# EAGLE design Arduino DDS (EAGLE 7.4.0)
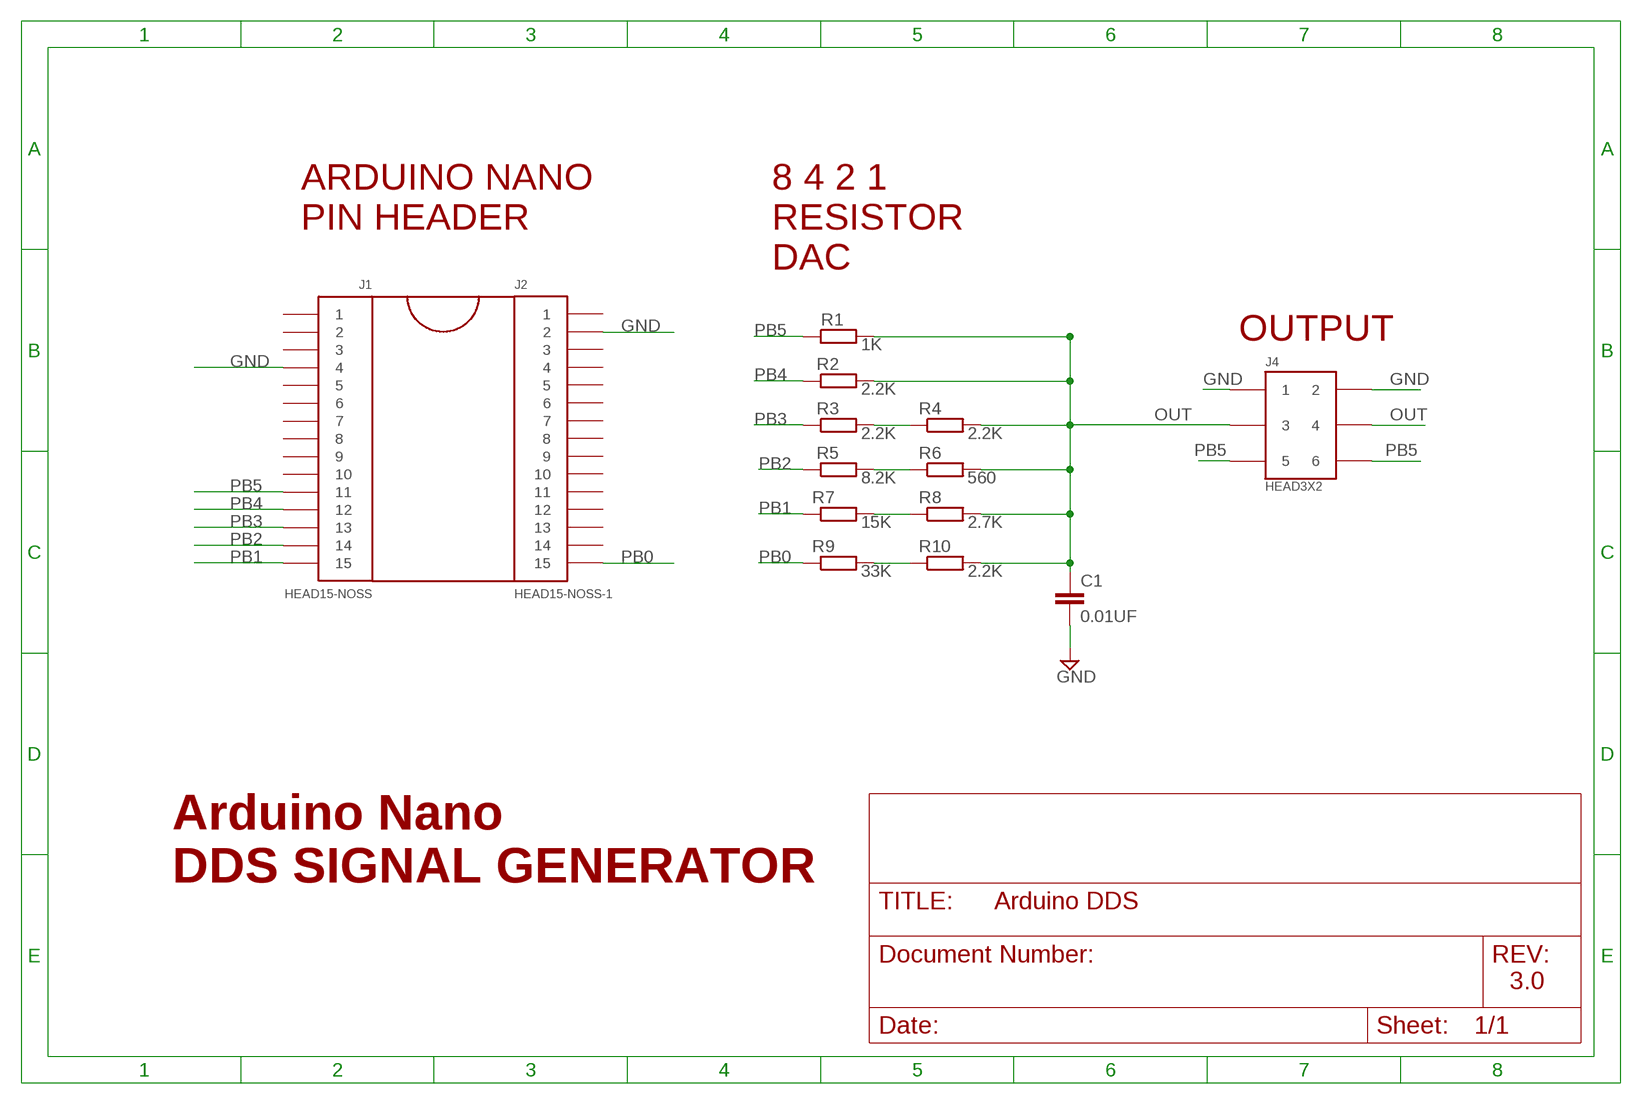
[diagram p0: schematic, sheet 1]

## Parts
C1  0.01UF  C-EUC0805  [C0805]
J1  HEAD15-NOSS  [HEAD15-NOSS]
J2  HEAD15-NOSS-1  [HEAD15-NOSS-1]
J4  HEAD3X2  [HEAD3X2]
R1  1K  R-EU_M0805  [M0805]
R2  2.2K  R-EU_M0805  [M0805]
R3  2.2K  R-EU_M0805  [M0805]
R4  2.2K  R-EU_M0805  [M0805]
R5  8.2K  R-EU_M0805  [M0805]
R6  560  R-EU_M0805  [M0805]
R7  15K  R-EU_M0805  [M0805]
R8  2.7K  R-EU_M0805  [M0805]
R9  33K  R-EU_M0805  [M0805]
R10  2.2K  R-EU_M0805  [M0805]

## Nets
GND: C1.2 J1.4 J2.2 J4.1 J4.2
N$7: R3.2 R4.1
N$8: R5.2 R6.1
N$9: R7.2 R8.1
N$10: R9.2 R10.1
OUT: C1.1 J4.3 J4.4 R1.2 R2.2 R4.2 R6.2 R8.2 R10.2
PB0: J2.15 R9.1
PB1: J1.15 R7.1
PB2: J1.14 R5.1
PB3: J1.13 R3.1
PB4: J1.12 R2.1
PB5: J1.11 J4.5 J4.6 R1.1
Unconnected: J1.1 J1.2 J1.3 J1.5 J1.6 J1.7 J1.8 J1.9 J1.10 J2.1 J2.3 J2.4 J2.5 J2.6 J2.7 J2.8 J2.9 J2.10 J2.11 J2.12 J2.13 J2.14

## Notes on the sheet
- ARDUINO NANO
  PIN HEADER
- 8 4 2 1
  RESISTOR
  DAC
- OUTPUT
- Arduino Nano
  DDS SIGNAL GENERATOR
- 3.0

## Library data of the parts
C1 = resistor:C-EU: CAPACITOR, European symbol
J1 = MyCON2:HEAD15-NOSS
J2 = MyCON2:HEAD15-NOSS-1
J4 = MyCON2:HEAD3X2
R1-R10 = resistor:R-EU_: RESISTOR, European symbol

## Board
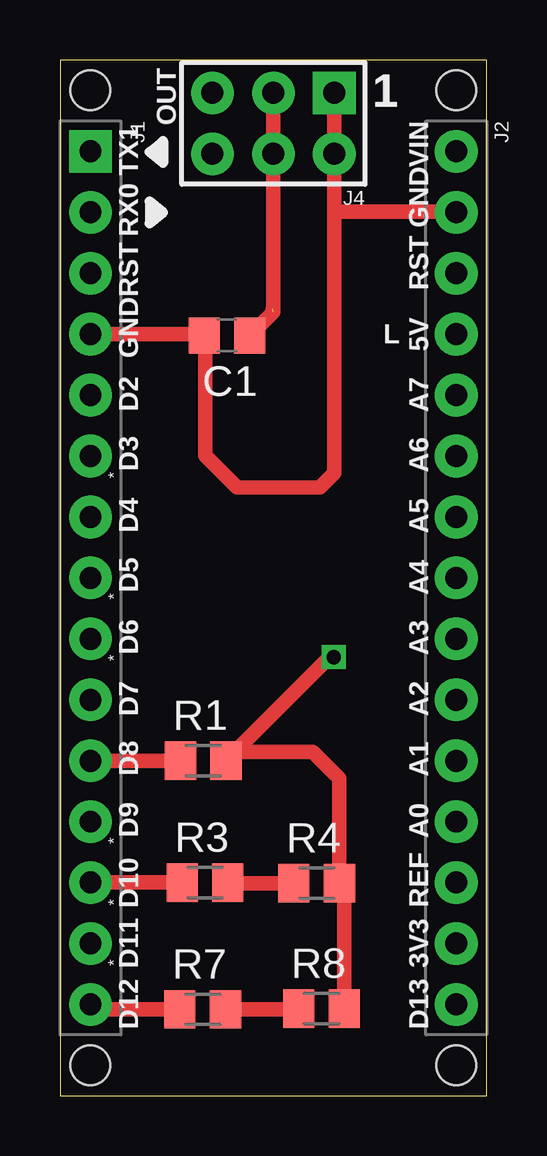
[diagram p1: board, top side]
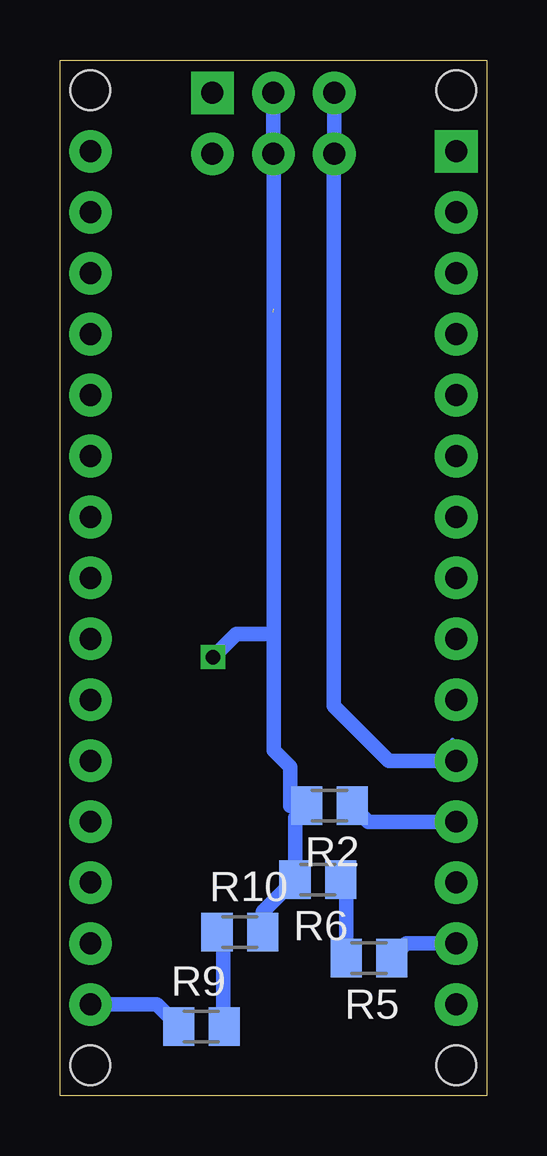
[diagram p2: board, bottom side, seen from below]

Size 17.78 x 43.18 mm. Coordinates in mm from the lower left corner, seen from the top.
Outline: 0,0 17.78,0 17.78,43.18 0,43.18 0,0
Copper layers (1*16): Top 0.035mm / dielectric 1.5mm / Bottom 0.035mm
Design rules "default *": minimum track width 8mil, minimum drill 16mil, track to track 8mil, track to pad 8mil, pad to pad 8mil, via to via 8mil, smd to smd 8mil, copper to edge 8mil, drill to drill 8mil, minimum pad ring 12mil, minimum via ring 8mil, stop-mask expansion 4mil, vias tented up to drill 18mil, thermal gap 10mil
Holes 1.65 mm at 1.27,1.27 16.51,1.27 16.51,41.91 1.27,41.91
tRestrict: area 0.1,0.1 to 2.4,2.4; area 15.4,40.8 to 17.7,43.1; area 15.4,0.1 to 17.7,2.4; area 0.1,40.8 to 2.4,43.1
bRestrict: area 15.4,0.1 to 17.7,2.4; area 0.1,0.1 to 2.4,2.4; area 0.1,40.8 to 2.4,43.1; area 15.4,40.8 to 17.7,43.1

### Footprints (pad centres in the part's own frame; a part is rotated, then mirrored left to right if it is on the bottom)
C0805 = smd 1.3 x 1.5: 1 -0.95,0; 2 0.95,0
HEAD15-NOSS = drill 0.914 pad 1.778 square: 1 0,0 | drill 0.914 pad 1.778: 2 2.54,0; 3 5.08,0; 4 7.62,0; 5 10.16,0; 6 12.7,0; 7 15.24,0; 8 17.78,0; 9 20.32,0; 10 22.86,0; 11 25.4,0; 12 27.94,0; 13 30.48,0; 14 33.02,0; 15 35.56,0
HEAD15-NOSS-1 = drill 0.914 pad 1.778: 1 0,0; 2 2.54,0; 3 5.08,0; 4 7.62,0; 5 10.16,0; 6 12.7,0; 7 15.24,0; 8 17.78,0; 9 20.32,0; 10 22.86,0; 11 25.4,0; 12 27.94,0; 13 30.48,0; 14 33.02,0; 15 35.56,0
HEAD3X2 = drill 0.914 pad 1.778 square: 1 0,0 | drill 0.914 pad 1.778: 2 0,2.54; 3 2.54,0; 4 2.54,2.54; 5 5.08,0; 6 5.08,2.54
M0805 = smd 1.3 x 1.6: 1 -0.95,0; 2 0.95,0

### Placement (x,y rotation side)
C1  6.96,31.7 180 top
J1  1.27,39.37 270 top
J2  16.51,39.37 270 top
J4  11.43,41.81 180 top
R1  5.97,13.97 0 top
R2  6.55,12.09 180 bottom
R3  6.05,8.89 0 top
R4  10.69,8.86 0 top
R5  4.9,5.74 180 bottom
R6  7.04,9.02 180 bottom
R7  5.94,3.61 0 top
R8  10.9,3.63 0 top
R9  11.89,2.9 0 bottom
R10  10.29,6.83 0 bottom

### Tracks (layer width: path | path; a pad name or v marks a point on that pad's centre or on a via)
GND
  Top 0.61: J1.4 6.01,31.75 C1.2 6.04,31.66 6.04,26.7 7.39,25.35 10.82,25.35 11.43,25.96 11.43,36.85 | J4.1 J4.2 11.43,36.85 | J2.2 16.48,36.85 11.43,36.85
N$7
  Top 0.61: R4.1 7,8.87 R3.2
N$8
  Bottom 0.61: R5.2 5.85,8.78 R6.1
N$9
  Top 0.61: R7.2 9.95,3.61 R8.1
N$10
  Bottom 0.203: 10.97,6.3 11.58,6.91 R10.1 | 10.97,3.05 R9.2
  Bottom 0.61: 10.97,3.05 10.97,6.57 R10.1
OUT  (via drill 0.6)  (1 unrouted)
  Top 0.61: R8.2 11.85,8.87 R4.2 11.64,13.22 10.53,14.33 7.28,14.33 | C1.1 8.89,32.68 J4.4 J4.3 | 8.87,32.79 8.89,32.82 | R1.2 7.28,14.33 | 7.28,14.33 11.24,18.29 v11.4,18.29
  Bottom 0.203: 7.32,11.99 R2.2 7.32,12.19 | 8.74,39.22 J4.4
  Bottom 0.61: J4.3 J4.4 | 8.74,39.22 8.87,39.09 8.87,19.25 | 8.87,19.25 8.87,14.4 8.18,13.72 8.18,12.09 R2.2 7.99,11.61 R6.2 9.34,7.67 R10.2 | v11.4,18.29 10.44,19.25 8.87,19.25
PB0
  Bottom 0.203: 13.01,3.05 R9.1
  Bottom 0.61: J2.15 13.75,3.81 R9.1
PB1
  Top 0.61: R7.1 1.27,3.61 J1.15
PB2
  Bottom 0.61: J1.14 3.34,6.35 R5.1
PB3
  Top 0.61: R3.1 J1.13
PB4
  Bottom 0.203: 5.08,11.99 R2.1
  Bottom 0.61: J1.12 4.94,11.43 R2.1
PB5
  Top 0.61: R1.1 J1.11
  Bottom 0.203: 1.42,14.83 1.42,14.02 J1.11 | 6.3,39.22 J4.6
  Bottom 0.61: J4.5 J4.6 | 6.3,39.22 6.38,39.22 6.38,16.26 4.09,13.97 J1.11

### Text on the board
tPlace: 1 | OUT | VIN | TX1 | RX0 | GND | RST | RST | GND | L | 5V | D2 | A7 | * | D3 | A6 | D4 | A5 | * | D5 | A4 | * | D6 | A3 | D7 | A2 | D8 | A1 | D9 | A0 | * | * | D10 | REF | * | D11 | 3V3 | D12 | D13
